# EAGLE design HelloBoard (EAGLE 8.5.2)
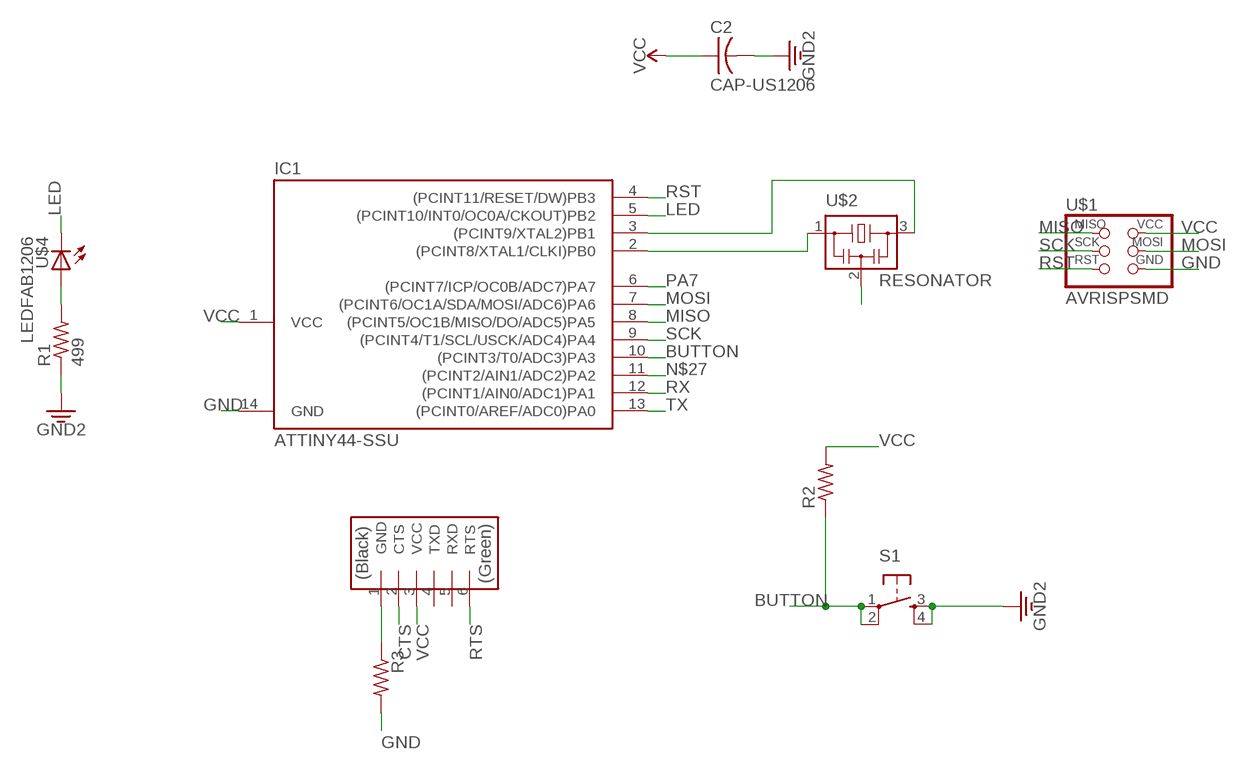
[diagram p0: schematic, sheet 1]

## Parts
C2  CAP-US1206  [C1206]
IC1  ATTINY44-SSU  [SOIC14]
R1  499  RES-US1206FAB  [R1206FAB]
R2  RES-US1206FAB  [R1206FAB]
R3  RES-US1206FAB  [R1206FAB]
S1  6MM_SWITCH6MM_SWITCH  [6MM_SWITCH]
U$1  AVRISPSMD  [2X03SMD]
U$2  RESONATOR  [EFOBM]
U$3  FTDI-SMD-HEADER  [1X06SMD]
U$4  LEDFAB1206  [LED1206FAB]

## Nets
BUTTON: IC1.10((PCINT3/T0/ADC3)PA3) R2.1 S1.1(P) S1.2(P1)
CTS: U$3.2(CTS)
GND: C2.2 IC1.14(GND) R1.1 R3.1 R3.2 S1.3(S) S1.4(S1) U$1.6(GND) U$2.2 U$3.1(GND) ; supply symbol labelled GND2
LED: IC1.5((PCINT10/INT0/OC0A/CKOUT)PB2) U$4.2(C)
MISO: IC1.8((PCINT5/OC1B/MISO/DO/ADC5)PA5) U$1.1(MISO)
MOSI: IC1.7((PCINT6/OC1A/SDA/MOSI/ADC6)PA6) U$1.4(MOSI)
N$1: IC1.2((PCINT8/XTAL1/CLKI)PB0) U$2.1
N$2: IC1.3((PCINT9/XTAL2)PB1) U$2.3
N$17: R1.2 U$4.1(A)
N$27: IC1.11((PCINT2/AIN1/ADC2)PA2)
PA7: IC1.6((PCINT7/ICP/OC0B/ADC7)PA7)
RST: IC1.4((PCINT11/RESET/DW)PB3) U$1.5(RST)
RTS: U$3.6(RTS)
RX: IC1.12((PCINT1/AIN0/ADC1)PA1)
SCK: IC1.9((PCINT4/T1/SCL/USCK/ADC4)PA4) U$1.3(SCK)
TX: IC1.13((PCINT0/AREF/ADC0)PA0)
VCC: C2.1 IC1.1(VCC) R2.2 U$1.2(VCC) U$3.3(VCC)
Unconnected: U$3.4(TXD) U$3.5(RXD)

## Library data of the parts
C2 = fab:CAP-US
IC1 = fab:ATTINY44
R1-R3 = fab:RES-US: Resistor (US Symbol)
S1 = fab:6MM_SWITCH: OMRON SWITCH
U$1 = fab:AVRISP
U$2 = fab:RESONATOR
U$3 = fab:FTDI-SMD-HEADER
U$4 = fab:LED: LED

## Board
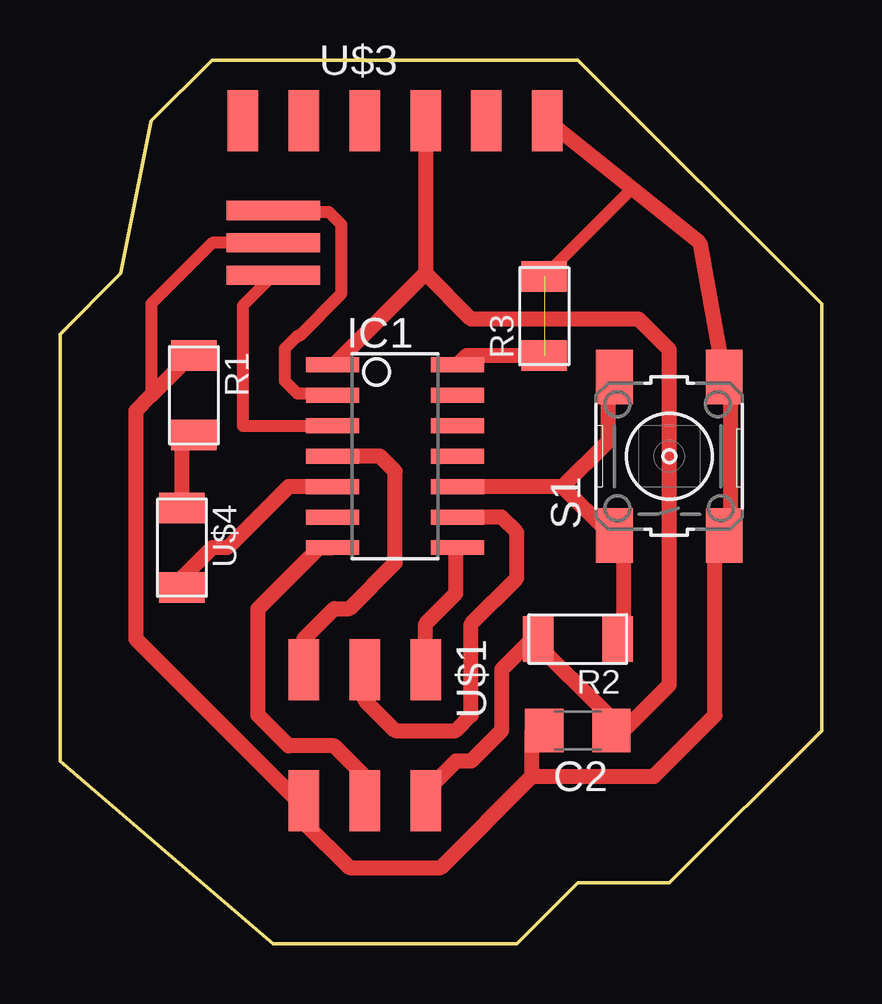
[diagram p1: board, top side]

Size 31.75 x 36.83 mm. Coordinates in mm from the lower left corner, seen from the top.
Outline: 0,7.62 8.89,0 19.05,0 21.59,2.54 25.4,2.54 31.75,8.89 31.75,26.67 21.59,36.83 6.35,36.83 3.81,34.29 2.54,27.94 0,25.4 0,7.62
Copper layers (1*16): Top 0.035mm / dielectric 1.5mm / Bottom 0.035mm
Design rules "default *": minimum track width 25mil, minimum drill 0.35mm, track to track 6mil, track to pad 25mil, pad to pad 25mil, via to via 6mil, smd to smd 15mil, copper to edge 15mil, drill to drill 6mil, minimum pad ring 10mil, minimum via ring 8mil, stop-mask expansion 4mil, vias tented up to drill 0mil, thermal gap 10mil

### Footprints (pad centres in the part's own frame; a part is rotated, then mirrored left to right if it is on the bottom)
C1206 = smd 1.6 x 1.8: 1 -1.4,0; 2 1.4,0
SOIC14 = smd 0.61 x 2.21: 1 -3.81,-2.603; 2 -2.54,-2.603; 3 -1.27,-2.603; 4 0,-2.603; 5 1.27,-2.603; 6 2.54,-2.603; 7 3.81,-2.603; 8 3.81,2.603; 9 2.54,2.603; 10 1.27,2.603; 11 0,2.603; 12 -1.27,2.603; 13 -2.54,2.603; 14 -3.81,2.603
R1206FAB = smd 1.27 x 1.905: 1 -1.651,0; 2 1.651,0
6MM_SWITCH = smd 2.286 x 1.524: 1 -3.302,2.286; 2 3.302,2.286; 3 -3.302,-2.286; 4 3.302,-2.286
2X03SMD = smd 2.54 x 1.27: 1 -2.54,2.54; 2 2.92,2.54; 3 -2.54,0; 4 2.92,0; 5 -2.54,-2.54; 6 2.92,-2.54
EFOBM = smd 0.8 x 3.9: 1 -1.35,0; 2 0,0; 3 1.35,0
1X06SMD = smd 2.54 x 1.27: 1 0,6.35; 2 0,3.81; 3 0,1.27; 4 0,-1.27; 5 0,-3.81; 6 0,-6.35
LED1206FAB = smd 1.27 x 1.905: 1 -1.651,0; 2 1.651,0

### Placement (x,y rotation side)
C2  21.59,8.89 180 top
IC1  13.97,20.32 270 top
R1  5.59,22.86 270 top
R2  21.59,12.7 180 top
R3  20.19,26.16 90 top
S1  25.4,20.32 90 top
U$1  12.7,8.89 270 top
U$2  8.89,29.21 270 top
U$3  13.97,34.29 270 top
U$4  5.08,16.51 270 top

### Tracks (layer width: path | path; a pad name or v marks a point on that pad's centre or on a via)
BUTTON
  Top 0.635: R2.1 23.5,12.7 23.5,16.51 S1.1 22.86,17.14 20.95,19.05 | 20.95,19.05 IC1.10 | 20.95,19.05 22.86,20.96 22.86,23.5 S1.2
GND  (1 unrouted)
  Top 0.508: U$2.2 6.35,29.21 3.81,26.67 3.81,22.86 | R3.2 23.82,31.44 23.88,31.44
  Top 0.635: U$3.1 23.88,31.44 26.67,29.21 S1.4 27.94,23.5 27.94,17.14 S1.3 27.3,16.51 27.3,9.53 24.77,6.99 19.68,6.99 | 19.68,6.99 19.68,8.89 C2.2 | 19.68,6.99 15.88,3.18 12.06,3.18 10.16,5.08 10.16,5.71 | 10.16,5.71 3.17,12.7 3.17,22.23 3.81,22.86 5.08,24.13 R1.1 | 10.16,5.71 U$1.6 | 20.32,27.94 R3.2 | R3.1 16.95,24.51 IC1.14
LED
  Top 0.635: IC1.5 9.53,19.05 6.99,16.51 6.35,16.51 5.08,15.24 U$4.2
MISO
  Top 0.635: U$1.1 15.24,13.34 16.51,14.61 16.51,16.51 IC1.8
MOSI
  Top 0.635: U$1.4 12.7,6.99 11.43,8.26 9.53,8.26 8.26,9.53 8.26,13.97 10.79,16.51 IC1.7
N$1
  Top 0.508: U$2.1 8.95,30.5 11.21,30.5 11.73,29.98 11.73,27.09 9.96,25.32 9.89,25.32 9.37,24.8 9.37,23.46 9.89,22.94 11.29,22.94 IC1.2
N$2
  Top 0.508: U$2.3 7.62,26.59 7.62,21.59 IC1.3
N$17
  Top 0.635: U$4.1 5.08,20.96 R1.2
RST
  Top 0.635: IC1.4 13.34,20.32 13.97,19.68 13.97,15.88 12.06,13.97 11.43,13.97 10.16,12.7 U$1.5
SCK
  Top 0.635: IC1.9 18.41,17.78 19.05,17.14 19.05,15.24 17.14,13.34 17.14,9.53 16.51,8.89 13.97,8.89 12.7,10.16 U$1.3
VCC
  Top 0.635: 15.24,27.94 11.43,24.13 IC1.1 | U$3.3 15.24,27.94 | 19.68,12.7 22.86,9.53 22.86,8.89 C2.1 23.5,8.89 25.4,10.79 25.4,24.77 24.13,26.04 17.14,26.04 15.24,27.94 | 19.68,12.7 18.41,11.43 18.41,8.89 17.14,7.62 16.51,7.62 15.24,6.35 U$1.2 | 19.68,12.7 R2.2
